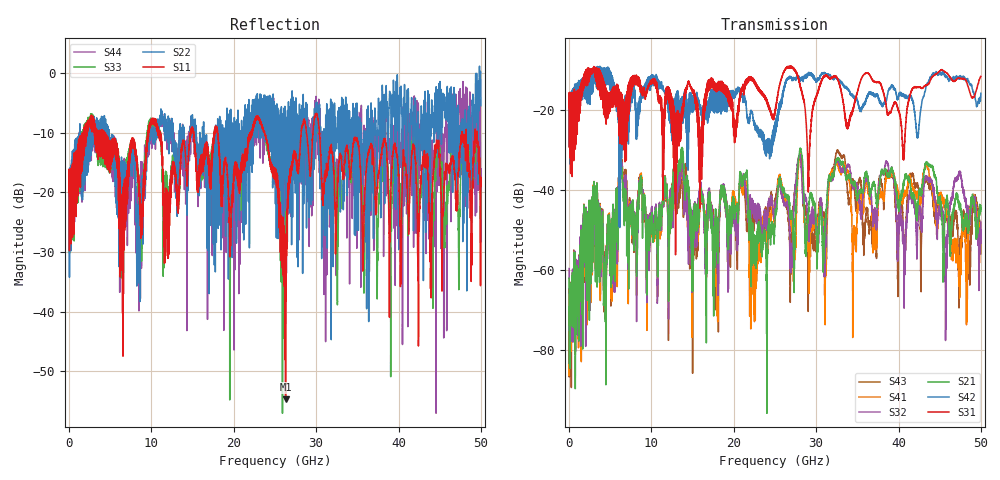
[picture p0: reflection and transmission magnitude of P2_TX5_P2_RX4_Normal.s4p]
!Keysight Technologies,N5225B,MY57041031,A.13.20.10
!Date: Friday, May 31, 2019 11:32:50
!Correction: S11(Full 4 Port(1,2,3,4))
!S12(Full 4 Port(1,2,3,4))
!S13(Full 4 Port(1,2,3,4))
!S14(Full 4 Port(1,2,3,4))
!S21(Full 4 Port(1,2,3,4))
!S22(Full 4 Port(1,2,3,4))
!S23(Full 4 Port(1,2,3,4))
!S24(Full 4 Port(1,2,3,4))
!S31(Full 4 Port(1,2,3,4))
!S32(Full 4 Port(1,2,3,4))
!S33(Full 4 Port(1,2,3,4))
!S34(Full 4 Port(1,2,3,4))
!S41(Full 4 Port(1,2,3,4))
!S42(Full 4 Port(1,2,3,4))
!S43(Full 4 Port(1,2,3,4))
!S44(Full 4 Port(1,2,3,4))
!S4P File: Measurements: <S11,S12,S13,S14>,
!<S21,S22,S23,S24>,
!<S31,S32,S33,S34>,
!<S41,S42,S43,S44>:
# Hz S  dB  R 50.0
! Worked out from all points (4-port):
!   5000 points, 10 MHz to 50 GHz, reference 50 ohm
!   strongest paths, dB at 10 MHz, 12.51 GHz, 25.01 GHz, 37.51 GHz, 50 GHz:
!     S31: -19.5, -17.8, -20.9, -13.2, -11.7
!     S42: -19.6, -27.8, -23.8, -16.7, -15.9
!     S21: -62.1, -44.4, -47.0, -42.8, -44.0
!     S32: -59.7, -43.6, -44.3, -41.9, -48.0
!     S41: -66.3, -44.2, -45.3, -44.6, -51.5
!     S43: -65.7, -43.0, -43.3, -40.8, -55.9
!   lowest |S11| = -54.7 dB at 26.29 GHz (marker M1), VSWR 1.00, Z = 50.1 - j0.177 ohm
!   |S11| at or under -10 dB: 4.282 GHz to 9.568 GHz (5.286 GHz wide, 76.3 % of centre); 23.74 GHz to 28.18 GHz (4.441 GHz wide, 17.1 % of centre); 30.39 GHz to 47.7 GHz (17.31 GHz wide, 44.3 % of centre)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
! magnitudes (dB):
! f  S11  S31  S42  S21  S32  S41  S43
! 10 MHz  -19.9  -19.5  -19.6  -62.1  -59.7  -66.3  -65.7
! 6.3 GHz  -27.4  -17.1  -23.5  -34.7  -33.3  -33.2  -32.3
! 22.88 GHz  -7.2  -14.7  -25.1  -50.6  -44.2  -50.6  -44.3
! 26.29 GHz  -54.7  -9.7  -13.3  -41.3  -44.0  -42.7  -44.1
! 30.01 GHz  -6.8  -16.7  -13.0  -51.0  -50.2  -51.2  -53.6
! 32.66 GHz  -18.2  -12.7  -12.6  -32.5  -32.9  -33.9  -30.3
! 50 GHz  -19.0  -11.7  -15.9  -44.0  -48.0  -51.5  -55.9
